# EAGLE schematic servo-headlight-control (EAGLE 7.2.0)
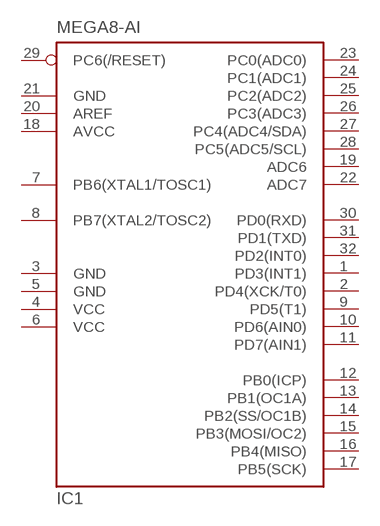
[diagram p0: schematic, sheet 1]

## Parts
IC1  MEGA8-AI  [TQFP32-08]
Unconnected: IC1.1(PD3(INT1)) IC1.2(PD4(XCK/T0)) IC1.7(PB6(XTAL1/TOSC1)) IC1.8(PB7(XTAL2/TOSC2)) IC1.9(PD5(T1)) IC1.10(PD6(AIN0)) IC1.11(PD7(AIN1)) IC1.12(PB0(ICP)) IC1.13(PB1(OC1A)) IC1.14(PB2(SS/OC1B)) IC1.15(PB3(MOSI/OC2)) IC1.16(PB4(MISO)) IC1.17(PB5(SCK)) IC1.19(ADC6) IC1.20(AREF) IC1.22(ADC7) IC1.23(PC0(ADC0)) IC1.24(PC1(ADC1)) IC1.25(PC2(ADC2)) IC1.26(PC3(ADC3)) IC1.27(PC4(ADC4/SDA)) IC1.28(PC5(ADC5/SCL)) IC1.29(PC6(/RESET)) IC1.30(PD0(RXD)) IC1.31(PD1(TXD)) IC1.32(PD2(INT0))

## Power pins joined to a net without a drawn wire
AVCC: IC1.18(AVCC)
GND: IC1.3(GND) IC1.5(GND) IC1.21(GND)
VCC: IC1.4(VCC) IC1.6(VCC)

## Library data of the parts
IC1 = atmel:MEGA8: MICROCONTROLLER 8 Kbytes FLASH, 1 kbytes SRAM, 512 bytes EEPROM, USART, 6-channel 10 bit ADC, 2-channel 8 bit ADC Pin compatible with Atmega48, ATMega88, ATMega168 Source: avr.lbr; MPN: ATMEGA8-16AU; OC_FARNELL: 9171371; OC_NEWARK: 73M8863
